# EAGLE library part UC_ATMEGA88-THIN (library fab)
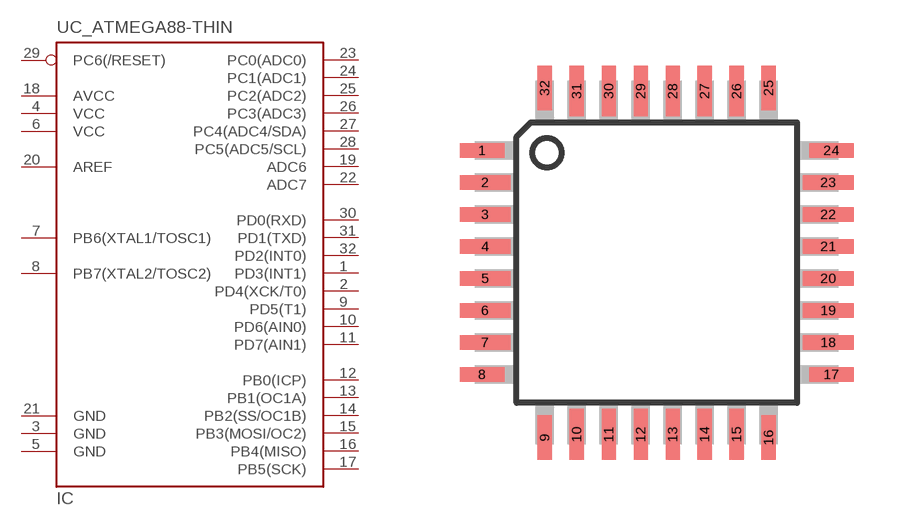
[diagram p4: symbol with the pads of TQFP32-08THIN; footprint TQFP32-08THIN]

Designator prefix IC

## UC_ATMEGA88-THIN  [TQFP32-08THIN]
1  PD3(INT1)
2  PD4(XCK/T0)
3  GND  pwr
4  VCC  pwr
5  GND  pwr
6  VCC  pwr
7  PB6(XTAL1/TOSC1)
8  PB7(XTAL2/TOSC2)
9  PD5(T1)
10  PD6(AIN0)
11  PD7(AIN1)
12  PB0(ICP)
13  PB1(OC1A)
14  PB2(SS/OC1B)
15  PB3(MOSI/OC2)
16  PB4(MISO)
17  PB5(SCK)
18  AVCC  pwr
19  ADC6
20  AREF  pas
21  GND  pwr
22  ADC7
23  PC0(ADC0)
24  PC1(ADC1)
25  PC2(ADC2)
26  PC3(ADC3)
27  PC4(ADC4/SDA)
28  PC5(ADC5/SCL)
29  PC6(/RESET)
30  PD0(RXD)
31  PD1(TXD)
32  PD2(INT0)

## Footprint TQFP32-08THIN (pad centres in mm)
smd 1.118 x 0.356: 1 -4.369,2.8; 8 -4.369,-2.8; 17 4.369,-2.8; 24 4.369,2.8
smd 1.27 x 0.356: 2 -4.293,2; 3 -4.293,1.2; 4 -4.293,0.4; 5 -4.293,-0.4; 6 -4.293,-1.2; 7 -4.293,-2; 18 4.293,-2; 19 4.293,-1.2; 20 4.293,-0.4; 21 4.293,0.4; 22 4.293,1.2; 23 4.293,2
smd 0.356 x 1.118: 9 -2.8,-4.369; 16 2.8,-4.369; 25 2.8,4.369; 32 -2.8,4.369
smd 0.356 x 1.27: 10 -2,-4.293; 14 1.2,-4.293; 15 2,-4.293; 26 2,4.293; 27 1.2,4.293; 31 -2,4.293
smd 0.35 x 1.27: 11 -1.2,-4.293; 12 -0.4,-4.293; 13 0.4,-4.293; 28 0.4,4.293; 29 -0.4,4.293; 30 -1.2,4.293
